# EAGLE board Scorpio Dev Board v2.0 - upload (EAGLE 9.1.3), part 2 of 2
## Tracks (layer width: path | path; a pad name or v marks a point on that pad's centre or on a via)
+5V  (via drill 0.48, 0.5, 0.8)
  Top 0.279: U1.73 59.42,28.71 v60.2,27.94
  Top 1.016: v85.85,20.19 85.85,19.68 90.04,15.49 JP12.1 JP12.2 JP12.3 JP12.4 | v5.59,87.63 56.46,87.63 57.98,86.19 57.98,80.45 68.45,69.98 73.53,69.98 79.63,63.88 79.63,61.72 79.76,61.59 82.96,61.59 84.84,59.72 U5.3 90.65,59.72 92.14,58.23 | X8.1 90.55,36.76 92.77,38.98 92.77,57.79 92.14,57.15 | 92.14,57.15 92.14,58.23 | R11.2 92.1,57.11 92.14,57.15 | JP14.2 92.33,55.88 92.33,58.42 | 92.33,58.42 92.14,58.23 | C12.1 92.33,60.68 92.33,58.42
  Bottom 0.61: v85.85,20.19 85.85,18.67 84.84,17.65 79.25,17.65 76.33,20.57 72.14,20.57 65.01,27.7 65.01,27.71 C9.1 62.09,27.94 v60.2,27.94
  Bottom 1.016: v85.85,20.19 85.85,35.79 X8.1 | JP5.1 6.22,82.68 3.68,85.22 R25.3 4.95,87.63 v5.59,87.63 5.59,90.3 6.1,90.81 8.64,90.81 9.91,92.08 JP20.2
AOUTL
  Top 0.254: U3.7 46.22,6.1 47.24,5.08 47.24,4.83 C39.1
AOUTR
  Top 0.254: U3.10 47.12,7.6 C38.1
BUTTON1
  Top 0.279: U1.29 31.33,32.22 21.34,22.22 JP15.12
  Bottom 0.305: 21.97,18.42 16.89,18.42
  Bottom 0.61: 21.97,18.42 22.61,19.05 22.61,21.59 21.97,22.22 JP15.12 | 16.89,18.42 16.19,19.11 15.91,19.39 15.24,19.39 12.29,19.39 R9.2 11.77,19.31 11.64,19.88 5.93,19.88 S2.3
BUTTON2
  Top 0.279: U1.34 32.89,29.71 21.59,18.42 19.43,18.42 JP15.13
BUTTON3
  Top 0.279: U1.87 71.98,35.72 73.28,34.42 74.04,34.42
  Top 0.305: 74.04,34.42 JP4.10 JP4.9
BUTTON4
  Top 0.279: U1.86 71.21,35.22 73.41,33.02 75.31,33.02 76.58,31.75
  Top 0.305: JP4.7 76.58,31.75
BUTTON5
  Top 0.279: U1.85 70.44,34.72 73.41,31.75
  Top 0.305: JP4.8 73.41,31.75
BUTTON6
  Top 0.279: U1.84 69.67,34.22 73.41,30.48 75.44,30.48
  Top 0.305: 75.44,30.48 JP4.5
BUTTON7
  Top 0.279: U1.83 68.9,33.72 73.41,29.21
  Top 0.305: JP4.6 73.41,29.21
CLKI  (via drill 0.5)
  Top 0.279: U1.71 55.62,24.89 57.15,23.37 57.28,23.37 | Y1.3 57.66,23.75 57.28,23.37 | v59.44,22.48 58.04,22.48 57.15,23.37 57.28,23.37
  Bottom 0.61: v59.44,22.48 62.61,22.48 65.53,19.56 JP10.1
CLKO  (via drill 0.5)
  Top 0.279: U1.72 56.12,25.67 56.39,25.4 v59.05,25.4
  Bottom 0.61: JP2.1 68.07,18.92 61.59,25.4 v59.05,25.4
D+  (via drill 0.5)
  Top 0.279: U1.77 63.14,30.71 64.52,29.34
  Top 0.406: 82.3,26.04 83.19,26.92 X1.D+
  Top 0.61: 64.52,29.34 72.9,20.96 80.39,20.96 80.77,21.34 v80.77,21.46 80.9,21.46 81.03,21.59 81.03,24.76 82.3,26.04
  Bottom 0.61: X8.3 86.68,41.4 82.68,41.4 81.15,39.88 81.15,21.84 v80.77,21.46
D-  (via drill 0.5)
  Top 0.279: U1.76 61.86,30.21 63.5,28.57
  Top 0.406: 83.57,25.4 83.57,25.65 84.19,26.27 X1.D-
  Top 0.61: 63.5,28.57 72.64,19.43 81.53,19.43 82.68,20.57 v82.68,21.46 82.68,24.51 83.57,25.4
  Bottom 0.61: X8.2 83.95,39.26 82.68,37.99 v82.68,21.46
DAC_FILT+
  Top 0.254: U3.6 45.47,5.6 C42.1
DAC_VQ
  Top 0.254: U3.5 40.69,4.62 40.26,4.19 40.26,4.17 C43.1
  Top 0.61: C43.1 C41.1
DEBUG_D+  (via drill 0.5)
  Top 0.254: X4.D+ 92.44,71.88 90.52,73.8 v90.39,73.8
  Bottom 0.406: v90.39,73.8 89.65,73.8 88.23,75.22 U11.15
DEBUG_D-  (via drill 0.5)
  Top 0.254: X4.D- 91.45,71.23 v90.42,72.26
  Bottom 0.406: U11.16 87.74,74.57 90.04,72.26 v90.42,72.26
DIPSW1
  Top 0.279: U1.27 29.79,33.22 21.34,24.76 JP15.10
DIPSW2
  Top 0.279: U1.28 30.56,32.72 21.34,23.5 19.43,23.5 JP15.9
ESP32_BOOT  (via drill 0.48, 0.5)
  Top 0.61: U6.25 96.14,81.92 94.87,83.19 v85.34,83.19 | v84.33,88.52 81.91,86.11 v81.91,84.2
  Top 0.813: v69.72,95.12 69.72,96.68 S4.2
  Bottom 0.61: v85.34,83.19 82.93,83.19 v81.91,84.2 | v84.33,88.52 v84.32,88.52 R30.1 80.86,88.69 77.85,88.69 74.97,91.57 70.1,91.57 69.72,91.95 v69.72,95.12
ESP32_CS  (via drill 0.48, 0.5)
  Top 0.279: U1.114 53.62,52.99 60.07,59.44 60.07,63.5 JP3.8
  Top 0.61: U6.29 93.47,87 v93.09,86.61 | v68.96,78.49 68.96,77.47 70.74,75.69 76.58,75.69 79.76,78.87 v81.28,78.87
  Bottom 0.61: JP3.8 58.8,67.31 68.96,77.47 v68.96,78.49 | v81.28,78.87 87.12,78.87 93.09,84.84 v93.09,86.61 93.09,89.41 R24.1
ESP32_EN  (via drill 0.5)
  Top 0.406: v77.09,93.22 76.64,93.22 75.56,92.13 75.56,89.53 75.06,89.03 71.37,89.03 70.17,87.82
  Top 0.61: U6.3 78.23,95.89 77.72,95.38 77.72,93.85 v77.09,93.22 | v69.09,81.28 69.09,86.79 70.17,87.82
  Bottom 0.61: R22.2 57.79,69.98 v69.09,81.28
  Bottom 0.813: R21.2 77.47,94.49 77.22,94.23 77.22,93.34 v77.09,93.22
ESP32_GPIO2  (via drill 0.48)
  Top 0.61: U6.24 94.36,78.89 93.57,78.11 v92.07,78.11
  Bottom 0.61: v92.07,78.11 93.6,79.63 R31.1
ESP32_HANDSHAKE  (via drill 0.5)
  Top 0.279: JP3.1 51.18,59.69 50.12,58.63 U1.121
  Top 0.61: U6.11 77.34,85.73 v77.28,85.66
  Bottom 0.305: JP3.1 52.45,63.5 | 52.45,63.5 | 52.45,66.55 52.45,63.5
  Bottom 0.61: 52.45,66.55 52.45,70.87 66.04,84.45 76.65,84.45 77.28,85.09 v77.28,85.66
ESP32_LED
  Top 0.61: U6.8 77.34,89.54 76.97,89.91 R23.1
ESP32_MISO  (via drill 0.48, 0.5)
  Top 0.279: U1.106 59.57,45.22 72.9,58.55 76.2,58.55 76.58,58.17 JP8.17
  Top 0.61: JP8.17 76.58,63.52 v71.9,68.2 | v75.6,78.49 77.25,78.49 79.16,80.39 v80.39,80.39 | v91.57,96.14 91.57,97.05 91.68,97.16 U6.37
  Bottom 0.406: 91.57,87.76 91.57,91.57
  Bottom 0.61: v75.6,78.49 75.6,75.58 71.9,71.88 v71.9,68.2 | v80.39,80.39 87,80.39 91.57,84.96 91.57,87.76 | 91.57,91.57 v91.57,96.14
ESP32_MOSI  (via drill 0.48, 0.5)
  Top 0.279: JP8.18 72.77,57.15 60.34,44.72 U1.105
  Top 0.61: v74.68,59.69 74.55,59.82 74.55,63.5 70.23,67.82 v70.23,68.2 | v73.8,78.49 73.8,82.69 73.79,82.71 v73.79,83.06 | v89.79,87.5 91.82,89.54 U6.31
  Bottom 0.61: JP8.18 74.68,57.79 v74.68,59.69 | v73.8,78.49 73.8,75.45 70.23,71.88 v70.23,68.2 | v89.79,87.5 87.5,87.5 85.6,85.6 81.53,85.6 78.99,83.06 v73.79,83.06
ESP32_MTDI
  Top 0.61: U6.14 76.98,81.92 76.21,81.15 R10.1
ESP32_RESET
  Top 0.279: U1.116 52.62,52.07 52.62,55.03 57.53,59.94 57.53,63.5 JP3.6
  Bottom 0.61: JP3.6 56.26,66.67 R22.1
ESP32_SCK  (via drill 0.48)
  Top 0.279: JP3.13 66.42,59.69 56.12,49.39 U1.109
  Top 0.61: v72.26,81.93 v72.26,78.49 | U6.30 92.71,88.27 89.92,85.47 v89.79,85.47
  Bottom 0.61: JP3.13 JP3.14 67.06,65.41 67.06,70.48 72.26,75.69 v72.26,78.49 | v89.79,85.47 85.98,81.66 72.53,81.66 v72.26,81.93
ESP32_TOUCH  (via drill 0.5, 0.8)
  Top 0.406: U6.9 79.52,88.14 72.26,88.14 v71.25,87.12
  Bottom 0.406: v71.25,87.12 68.45,87.12 v67.56,88.01
ESP32_VDD  (via drill 0.5)
  Top 0.61: 82.04,96.65 89.53,96.65 v90.04,96.14
  Top 0.813: U6.2 81.53,97.16 82.04,96.65 v82.04,96.27
  Top 0.914: C25.+ 75.92,97.16 U6.2
  Top 1.27: U7.2 U7.4 59.97,93.75 C33.1 64.24,93.75 64.52,93.47 74.17,93.47 75.67,94.97 C25.+
  Bottom 0.61: R30.2 C36.1 | R24.2 90.04,89.66 v90.04,96.14 90.04,96.39
  Bottom 0.813: C35.1 83.72,91.44 C36.1 | R21.1 82.04,95.29 v82.04,96.27
  Bottom 1.016: R21.1 82.43,93.85 C35.1 83.72,95.73 83.57,95.89 82.42,95.89 v82.04,96.27 82.57,95.73
ESP32_WAKE  (via drill 0.5)
  Top 0.279: JP3.5 56.26,59.69 54.36,57.79 52.12,55.55 U1.117
  Top 0.61: U6.10 73.28,87 70.61,84.33 v70.61,78.47
  Bottom 0.279: JP3.5 56.26,62.48 57.28,63.5 59.82,63.5 60.07,63.75 60.07,66.55
  Bottom 0.61: v70.61,78.47 70.61,77.34 60.07,66.8 60.07,66.55
FLASH_CS
  Top 0.279: U1.53 46.62,25.58 46.62,19.06 43.69,16.13 JP19.9
  Bottom 0.61: JP19.9 43.69,14.86 43.43,15.11 41.27,17.27 U2.1
FLASH_HOLD
  Top 0.279: JP19.5 48.77,14.73 49.12,15.08 49.12,25.58 U1.58 | JP19.5
FLASH_MISO
  Top 0.279: U1.48 44.12,21.26 40.51,17.65 40.39,17.65 38.48,17.65 37.34,16.51 37.34,13.21 JP19.14
  Bottom 0.305: 37.34,16 37.34,13.21 JP19.14
  Bottom 0.61: 37.34,16 37.34,19.43 40.39,22.48 U2.2
FLASH_MOSI
  Top 0.279: U1.69 54.62,23.36 60.2,17.78 60.2,14.48 60.2,13.21 JP7.2
  Bottom 0.61: U2.5 53.09,25.02 62.99,15.11 62.99,13.46 JP7.2
FLASH_SCK
  Top 0.279: JP19.6 47.5,13.21 47.5,15.24 48.62,16.36 48.62,25.58 U1.57
  Bottom 0.305: JP19.6 50.04,13.21 50.04,15.49 51.18,16.64
  Bottom 0.61: 51.18,16.64 51.18,23.24 50.67,23.75 U2.6
FLASH_WP
  Top 0.279: U1.47 43.62,21.65 40.64,18.67 38.23,18.67 36.07,16.51 JP19.15
  Bottom 0.61: JP19.15 36.07,18.54 | 36.07,18.54 36.07,20.19 39.62,23.75 U2.3 | R32.2 36.07,18.54
LCD_CS  (via drill 0.5)
  Top 0.279: U1.21 25.17,36.22 21.34,32.39 JP15.4
  Top 0.305: JP5.4 8.64,83.95 8.64,81.28
  Top 0.61: v7.87,76.33 8.64,77.09 8.64,81.28
  Bottom 0.305: JP15.4 22.48,32.39 22.99,32.89 22.99,35.81 22.61,36.2 16.89,36.2
  Bottom 0.61: 16.89,36.2 16.38,36.2 14.99,37.59 14.99,38.73 7.24,46.48 7.24,74.8 7.24,75.69 v7.87,76.33
LCD_RESET
  Top 0.279: U1.8 30.06,42.72 21.34,51.44 19.43,51.44 JP6.7
  Top 0.305: 13.72,80.9 13.72,83.95 JP5.8
  Top 0.61: 13.72,80.9 13.72,55.5 16.51,52.7 JP6.7
LCD_TE
  Top 0.279: U1.2 34.68,45.72 21.34,59.06 19.43,59.06 JP6.1
  Top 0.61: JP6.1 14.99,63.5 JP5.7
LED1
  Top 0.279: JP19.20 JP19.19 31.11,14.61 31.11,16.38 36.7,21.97 38.99,21.97 39.24,22.22 41.62,24.6 U1.43
  Top 0.305: R13.1 27.18,10.03 27.56,10.41 29.84,10.41 30.99,11.56
  Top 0.61: 30.99,11.56 JP19.20
LED2
  Top 0.279: U1.44 42.12,23.96 39.5,21.34 37.34,21.34 32.26,16.26 32.26,14.1 | JP19.18 32.26,13.21
  Top 0.305: 32.26,14.1 32.26,13.21 | R16.1 30.73,9.02 30.73,10.03 31.11,10.41 32.89,10.41 33.53,11.05 JP19.18
LED3  (via drill 0.48)
  Top 0.279: U1.45 42.62,23.19 | 42.62,23.19 | 42.62,23.19 40.01,20.57 37.85,20.57 33.53,16.26 JP19.17
  Top 0.305: R12.1 34.8,9.78 v34.8,10.54
  Bottom 0.305: v34.8,10.54 34.8,12.7 33.53,13.97 JP19.17
LED4
  Top 0.279: U1.46 43.12,22.42 40.26,19.56 37.85,19.56 34.8,16.51 34.8,13.21 JP19.16
  Top 0.305: R27.1 37.21,10.8 JP19.16
MCLR  (via drill 0.5)
  Top 0.279: U1.20 24.4,36.72 21.34,33.66 19.43,33.66 JP15.1
  Top 0.406: JP22.6 4.06,8.38 4.06,13.97 4.06,17.27 5.08,18.29 6.6,18.29 7.75,17.14 9.02,17.14 9.02,17.15
  Top 0.61: v11.68,30.1 11.68,22.99 9.27,20.57 R1.2 9.02,17.15
  Bottom 0.305: 16.89,31.11 19.05,31.11 19.43,31.5 19.43,33.66 JP15.1
  Bottom 0.61: v11.68,30.1 15.49,30.1 16.51,31.11 16.89,31.11
MCLR_IN
  Top 0.61: S1.3 5.82,11.28 6.61,12.07 R2.2 R1.1 11.91,14.35 C10.1
MCU_VDD  (via drill 0.5, 0.8)
  Top 0.279: 52.83,45.08 52.83,37.23 52.84,37.22 | v39.37,43.69 42.12,46.44 U1.137 | v51.94,45.72 50.55,45.72 49.62,46.64 U1.122 | U1.107 54.86,45.72 v54.74,45.72 | U1.88 v54.74,36.22 | U1.74 54.73,29.21 v54.1,29.85 | U1.33 38.11,30.21 38.48,29.85 v38.48,29.59 | U1.18 40.39,37.72 v41.27,36.83 | U1.55 47.62,29.21 v48.26,29.85 | U1.64 52.12,29.54 v51.82,29.85 | U1.41 40.62,29.06 v41.15,29.59
  Top 0.406: 57.75,48.86 57.28,48.39 57.28,47.37 55.63,45.72 54.86,45.72
  Top 0.61: v54.74,36.22 53.85,36.22 52.84,37.22 52.84,45.08 52.83,45.08 52.32,45.59 52.32,45.72
  Top 1.016: 57.75,48.86 68.07,59.18 v68.96,59.18 | v54.74,45.72 52.32,45.72 v51.94,45.72
  Bottom 0.61: C8.1 v54.74,45.72 | v51.94,45.72 C7.1 51.69,43.66 41.4,43.66 C6.1 | C1.1 41.55,36.55 v41.27,36.83 38.25,33.81 C2.1 38.25,29.82 v38.48,29.59 | v41.15,29.59 43.26,29.59 C4.1 47.01,28.6 v48.26,29.85 | R32.1 32.23,18.61 28.7,18.61 | 28.7,18.61 28.26,18.61 | v48.26,29.85 v51.82,29.85 52.2,30.23 C22.1 | C5.1 v48.26,29.85 | 54.12,29.83 54.12,35.59 v54.74,36.22 56.9,36.22 57.66,35.45 C3.1 | 28.7,18.61 28.13,18.61 26.29,16.76 25.78,16.76 21.21,12.19 L6.1 | C21.1 53.74,27.81 53.74,27.89 54.1,28.68 v54.1,29.85
  Bottom 0.813: v51.82,29.85 v54.1,29.85 54.12,29.83 | v39.37,43.69 41.17,43.69 C6.1
  Bottom 1.016: L3.1 71.65,62.38 68.96,59.69 v68.96,59.18 | 28.26,18.61 38.48,28.83 v38.48,29.59 v41.15,29.59
MISO4
  Top 0.279: JP8.12 72.77,49.53 64.96,41.72 U1.99
MOSI4
  Top 0.279: U1.104 61.11,44.22 66.17,49.28 72.77,55.88 75.31,55.88 JP8.15
N$1
  Top 0.61: R25.2 1.14,95.38 2.29,96.52 11.56,96.52 12.45,95.63 JP20.3
N$2
  Top 0.61: LED3.A R12.2
N$3
  Top 0.61: R23.2 72.03,90.81 LED6.A
N$6
  Top 0.61: C26.1 6.12,50.88 R19.2 C20.2
N$7
  Top 0.61: LED4.A 37.21,4.99 R27.2
  Top 1.016: LED4.A
N$8
  Bottom 0.61: R28.1 R29.1 20.03,38.14 JP13.1
N$11
  Bottom 0.406: R20.2 49.02,46.57 U8.2
N$12
  Bottom 1.016: JP23.1 84.58,10.17 X9.TSH
N$14
  Bottom 0.406: U8.1 50.29,51.44
  Bottom 0.61: 50.29,51.44 R4.2
N$15
  Bottom 0.406: U8.3 47.75,48.64 47.5,48.39 R7.2
N$17
  Top 1.016: R11.1 90.04,52.93 89.69,52.58 LED5.A
N$19
  Bottom 0.406: R8.1 37.72,57.28 39.24,55.75 46.02,55.75 U8.5
N$20
  Bottom 1.016: JP25.1 79.5,10.25 X9.RSH
N$21
  Bottom 0.406: U8.6 47.75,58.8 47.37,59.18 R17.1
N$22
  Bottom 0.61: X9.TIP 87.42,8.81 86.61,8 70.1,8 68.07,10.03 X3.3
N$23
  Bottom 0.61: X9.RING 77.25,9.65 70.74,9.65 70.06,10.33 X3.2
N$24  (via drill 0.48)
  Top 0.406: v84.2,73.91 83.03,73.91 C16.1
  Bottom 0.406: U11.17 v84.2,73.91
N$25
  Top 1.27: C28.1 48.64,93.07 U7.3 54.89,93.07 57.66,90.3 JP24.1
N$26
  Top 0.61: C18.2 5.56,57.28 C23.1 6.2,57.71 R15.2
N$27
  Top 0.61: R13.2 LED1.A
N$31
  Bottom 0.406: U8.7 49.02,60.07 48.26,60.83 45.47,60.83 45.21,60.58 45.21,57.66 44.7,57.15 41.02,57.15 R18.1
N$32
  Bottom 0.61: L3.2 74.65,64.69 C15.1
  Bottom 1.016: L3.2 L1.2
N$33
  Bottom 1.016: L5.2 17.19,12.55 L6.2 17.68,12.07 C17.1
N$34
  Top 0.61: X3.4 66.08,4.87 65.91,4.7 C40.1 59.03,2.92 58.27,2.16 R42.1
N$35
  Top 0.61: C39.2 50.65,2.39 R41.1 52.7,2.29 R42.2
N$38
  Top 0.61: C38.2 R39.2 54.73,9.53 R40.2
N$39
  Top 0.61: X3.5 64.07,7.68 63.37,6.98 C37.1 59.03,9.43 R40.1
N$46  (via drill 0.48)
  Top 0.406: v89.37,66.26 92.38,63.25 TX.C
  Bottom 0.406: R14.2 89.17,66.46 v89.37,66.26
N$63  (via drill 0.48)
  Top 0.406: v90.68,69.09 91.82,67.95 91.82,67.82 91.82,66.93 93.22,65.53 RX.C
  Bottom 0.406: R38.2 90.68,70.45 v90.68,69.09
N$80
  Top 0.61: LED2.A R16.2
OC2  (via drill 0.5)
  Top 0.279: U1.11 27.75,41.22 21.34,47.62 JP6.12
  Top 0.61: R19.1 10.95,48.9 v11.05,48.9
  Bottom 0.305: JP6.12 19.43,48.9 16.76,48.9
  Bottom 0.61: 16.76,48.9 v11.05,48.9
OC6  (via drill 0.5)
  Top 0.279: U1.6 31.6,43.72 21.34,53.98 19.43,53.98 JP6.5
  Top 0.61: R15.1 v10.92,55.25
  Bottom 0.61: JP6.5 v10.92,55.25
PGEC
  Top 0.279: U1.35 33.53,29.21 21.46,17.14 JP15.16
  Top 0.61: JP15.16 20.7,12.32 17.91,9.53 16.26,7.87 JP22.2
PGED  (via drill 0.5)
  Top 0.279: U1.36 34.05,28.71 25.4,20.07 v25.4,19.56
  Top 0.305: JP15.15 18.16,17.02
  Top 0.61: 18.16,17.02 18.16,15.24 18.16,12.45 13.84,8.13 13.84,6.48 JP22.3
  Bottom 0.406: v25.4,19.56 21.34,15.49 18.67,15.49 18.16,16 JP15.15
PMA0  (via drill 0.5)
  Top 0.279: U1.30 32.1,31.71 21.34,20.96 19.43,20.96 JP15.11
  Top 0.61: v14.35,34.42 14.86,34.42 15.62,33.66 15.62,24.89 18.16,22.35 JP15.11
  Bottom 0.305: JP5.3 8.64,83.95 8.64,87.38
  Bottom 0.61: v14.35,34.42 13.72,35.05 13.72,37.59 4.83,46.48 4.3,47.01 4.3,64.84 3.43,65.71 3.43,70.23 4.38,71.18 4.38,76.01 9.91,81.53 JP5.3 | JP20.4 15.11,94.11 15.11,90.93 12.32,88.14 9.4,88.14 8.64,87.38
PMCS1
  Top 0.279: JP8.10 72.77,46.99 66.5,40.72 U1.97
PMD0
  Top 0.279: U1.135 43.12,54.03 35.94,61.21 JP9.9
  Bottom 0.305: 16.26,81.15 16.26,83.95 JP5.10
  Bottom 0.61: JP9.9 34.42,60.71 25.02,60.71 23.88,61.85 23.88,63.63 21.46,66.04 19.94,66.04 16.26,69.72 16.26,81.15
PMD1
  Top 0.279: JP9.8 JP9.7 33.4,61.59 35.18,59.82 36.2,59.82 41.62,54.39 U1.138
  Bottom 0.61: JP5.9 17.53,75.95 22.92,70.55 25.78,70.55 25.78,70.48 28.96,67.31 32.77,67.31 33.4,66.67 JP9.8
PMD2  (via drill 0.5)
  Top 0.279: U1.142 39.62,50.29 33.65,56.26 32.38,56.26 28.32,60.33 JP9.3
  Top 0.305: 18.8,81.03 18.8,83.44 18.8,83.95 JP5.12
  Top 0.61: 18.8,81.03 18.8,80.65 v18.8,70.48
  Bottom 0.305: 27.05,66.42 27.05,63.5 JP9.3
  Bottom 0.61: v18.8,70.48 20.07,69.22 24.51,69.22 27.05,66.67 27.05,66.42
PMD3  (via drill 0.5)
  Top 0.279: JP9.2 27.05,63.5 27.05,60.33 31.75,55.63 33.27,55.63 39.12,49.78 U1.143
  Top 0.61: JP9.2 25.78,66.93 25.15,67.56 v25.15,72.39
  Bottom 0.61: JP5.11 20.07,75.95 23.62,72.39 v25.15,72.39
PMD4
  Top 0.279: JP9.1 25.78,60.33 31.11,54.99 32.89,54.99 38.62,49.26 U1.144
  Top 0.305: JP5.14 23.88,83.95 23.88,81.03
  Top 0.61: JP9.1 23.88,64.14 23.88,81.03
PMD5  (via drill 0.5)
  Top 0.279: U1.3 33.91,45.22 21.34,57.79 JP6.4
  Top 0.61: JP5.13 22.61,66.67 22.35,66.42 v22.35,62.74
  Bottom 0.61: v22.35,62.74 22.48,62.61 22.48,58.67 21.59,57.79 JP6.4
PMD6  (via drill 0.5)
  Top 0.279: U1.4 33.14,44.72 21.34,56.52 19.43,56.52 JP6.3
  Top 0.61: v19.3,62.87 20.83,64.39 20.83,76.2 v21.34,76.71
  Bottom 0.305: 23.88,81.03 23.88,83.95 JP5.16
  Bottom 0.61: v21.34,76.71 23.88,79.25 23.88,81.03 | JP6.3 16.51,57.79 15.75,58.55 15.75,61.98 16.64,62.87 v19.3,62.87
PMD7
  Top 0.279: U1.5 32.37,44.22 21.34,55.25 JP6.6
  Bottom 0.305: 37.21,60.58 37.21,66.42
  Bottom 0.61: 37.21,60.58 36.2,59.56 27.05,59.56 22.73,55.25 JP6.6 | JP5.15 25.15,78.23 27.05,76.33 27.05,72.39 30.23,69.22 34.42,69.22 37.21,66.42
PMD8
  Top 0.279: U1.128 46.62,51.44 46.62,59.17 44.83,60.96 44.83,63.5 JP9.16
  Top 0.305: 26.42,81.03 26.42,83.95 JP5.18
  Top 0.61: 26.42,81.03 26.42,77.09 35.94,67.56 42.93,67.56 43.56,66.93 JP9.16
  Bottom 0.61: JP20.7 22.61,89.15 24.07,87.69 26.61,87.69 27.69,86.61 JP5.18
PMD9  (via drill 0.5)
  Top 0.279: U1.127 47.12,59.94 46.1,60.96 JP9.17
  Top 0.61: JP5.17 27.69,77.6 36.58,68.71 44.32,68.71 44.83,68.2 v44.83,66.8
  Bottom 0.305: v44.83,66.8 44.83,63.5 JP9.17 | JP5.17 28.96,83.95 28.96,87.12
  Bottom 0.61: 28.96,87.12 27.43,88.65 25.4,88.65 25.15,88.9 JP20.8
PMD10  (via drill 0.5)
  Top 0.279: U1.125 48.12,59.17 48.64,59.69 JP9.19
  Top 0.305: JP5.20 28.96,83.95 28.96,81.03
  Top 0.61: v47.37,66.8 47.37,68.33 45.85,69.85 37.21,69.85 28.96,78.11 28.96,81.03
  Bottom 0.305: v47.37,66.8 47.37,63.5 JP9.19
  Bottom 0.61: JP5.20 30.1,85.34 30.1,87.25 27.69,89.66 JP20.9
PMD11
  Top 0.279: U1.124 48.62,58.4 49.91,59.69 49.91,63.5 JP9.20
  Top 0.61: JP5.19 30.23,78.74 37.97,70.99 47.5,70.99 48.64,69.85 JP9.20
  Bottom 0.305: JP5.19 31.5,83.95 31.5,87
  Bottom 0.61: 31.5,87 31.5,88.65 30.86,89.28 30.35,89.28 30.23,89.41 JP20.10
PMD12
  Top 0.279: JP3.10 62.61,63.5 62.61,59.69 54.62,51.7 U1.112
  Top 0.305: JP5.22 32.77,85.09 31.5,83.82 31.5,81.03
  Top 0.61: JP3.10 61.34,67.37 60.71,68.01 52.39,68.01 48.26,72.14 38.86,72.14 31.94,79.06 31.5,79.5 31.5,81.03
  Bottom 0.61: JP5.22 32.77,88.9 JP20.11
PMD13  (via drill 0.5)
  Top 0.279: JP3.9 61.34,59.69 54.12,52.47 U1.113
  Top 0.61: JP5.21 32.77,79.88 39.31,73.34 49.59,73.34 53.59,69.34 61.59,69.34 62.61,68.33 v62.61,66.8
  Bottom 0.305: JP3.9 62.61,63.5 v62.61,66.8 | JP5.21 34.04,83.95 34.04,87
  Bottom 0.61: 34.04,87 34.04,89.28 35.31,90.55 JP20.12
PMD14
  Top 0.279: U1.110 55.62,50.16 65.15,59.69 65.15,63.5 JP3.12
  Top 0.305: JP5.24 34.04,83.95 34.04,81.03
  Top 0.61: JP3.12 63.88,68.71 62.1,70.48 54.36,70.48 50.42,74.42 40.13,74.42 34.04,80.52 34.04,81.03
  Bottom 0.305: JP5.24 35.31,87.12 | 35.31,88.27 35.43,88.39
  Bottom 0.61: 35.31,87.12 35.31,88.27 | JP20.13 37.85,90.81 35.43,88.39
PMD15  (via drill 0.5)
  Top 0.279: U1.111 55.12,50.93 63.88,59.69 JP3.11
  Top 0.61: JP5.23 35.31,81.28 41.02,75.56 51.18,75.56 55.12,71.63 62.74,71.63 65.15,69.22 v65.15,68.45
  Bottom 0.305: JP3.11 65.15,63.5 v65.15,68.45 | JP5.23 36.58,83.95 36.58,87.12
  Bottom 0.61: JP20.14 40.39,91.44 36.58,87.63 36.58,87.12
PMRD
  Top 0.279: U1.13 26.21,40.22 21.34,45.08 JP6.14
  Bottom 0.279: JP6.14 20.7,45.72
  Bottom 0.305: 20.7,45.72 20.07,46.36 16.89,46.36 | JP5.6 11.18,83.95 11.18,81.15
  Bottom 0.61: 16.89,46.36 11.05,46.36 8.89,48.51 8.89,74.93 11.18,77.22 11.18,81.15
PMWR
  Top 0.279: U1.12 26.98,40.72 21.34,46.36 19.43,46.36 JP6.11
  Top 0.61: JP6.11 17.14,47.62 12.45,52.32 JP5.5
  Bottom 0.305: JP5.5 13.72,83.95 13.72,87.63
  Bottom 0.61: 13.72,87.63 14.35,88.27 18.16,88.27 20.07,90.17 JP20.6
PWM_OC2
  Top 0.406: C26.2 8.99,52.83 7.87,52.83 7.62,53.09 7.62,56.39 10.59,59.36 X6.TIP
PWM_OC6
  Top 0.61: C23.2 8.25,62.97 8.25,72.14 9.02,72.9 10.51,72.9 X6.RING
RA1
  Top 0.279: JP19.8 JP19.7 46.23,13.34 46.23,15.24 48.12,17.13 48.12,25.58 U1.56
RA9
  Top 0.279: JP1.2 27.18,11.94 27.05,12.07 27.05,15.24 35.18,23.37 35.56,23.37 37.72,23.37 39.62,25.27 U1.39
RA10
  Top 0.279: U1.40 40.12,24.88 37.97,22.73 35.56,22.73 28.32,15.49 JP1.1
RB4
  Top 0.279: U1.26 29.02,33.72 21.34,26.04 19.43,26.04 JP15.7
RB6
  Top 0.279: JP1.4 24,11.94 23.88,12.07 23.88,15.24 35.48,26.85 U1.37
RB7
  Top 0.279: U1.38 39.12,25.78 37.46,24.13 34.67,24.13 25.78,15.24 JP1.3
RB11
  Top 0.279: U1.50 45.12,20.45 40.68,16 40.39,16 39.88,15.49 39.88,13.21 JP19.12
RB12
  Top 0.279: U1.59 49.62,16.61 50.04,16.19 50.04,13.21 JP19.4
RB13
  Top 0.279: U1.60 50.12,17.32 51.31,16.13 JP19.3
RE8
  Top 0.279: U1.23 26.71,35.22 21.34,29.85 JP15.6
RE9
  Top 0.279: U1.24 27.48,34.72 21.34,28.57 19.43,28.57 JP15.5
REFCLKO1  (via drill 0.5)
  Top 0.254: U3.4 39.51,6.1 v39.12,5.71
  Top 0.279: U1.70 55.12,23.87 61.59,17.4 61.59,14.61 JP7.1
  Bottom 0.279: JP7.1 60.2,13.21 60.2,9.4 59.69,8.89 57.66,8.89
  Bottom 0.61: 57.66,8.89 55.75,6.98 52.7,6.98 51.43,5.71 v39.12,5.71
RF4
  Top 0.279: U1.90 71.5,37.22 72.01,37.22 73.66,37.22 JP8.2
RF5
  Top 0.279: JP8.1 75.31,38.1 72.77,38.1 72.39,37.72 U1.91
RG15
  Top 0.279: U1.1 35.57,46.22 21.46,60.33 JP6.2
RH4
  Top 0.279: U1.65 52.62,20.02 55.12,17.53 55.12,13.21 JP7.6
RH5
  Top 0.279: U1.66 53.12,20.92 56.39,17.65 JP7.5
RH6
  Top 0.279: U1.67 53.62,21.94 57.66,17.91 57.66,13.21 JP7.4
RH7
  Top 0.279: U1.68 54.12,22.71 58.93,17.91 JP7.3
RH8
  Top 0.279: U1.81 67.36,32.72 73.41,26.67
  Top 0.305: JP4.4 73.41,26.67
RH9
  Top 0.279: U1.82 68.13,33.22 73.41,27.94 75.44,27.94
  Top 0.305: 75.44,27.94 JP4.3
RH12
  Top 0.279: JP8.11 75.31,50.8 72.77,50.8 64.19,42.22 U1.100
RH13
  Top 0.279: U1.101 63.42,42.72 72.77,52.07 JP8.14
RH14
  Top 0.279: JP8.13 75.31,53.34 72.77,53.34 62.65,43.22 U1.102
RJ4
  Top 0.279: JP9.11 38.48,61.09 43.62,55.94 44.12,55.45 U1.133
RJ7
  Top 0.279: U1.134 43.62,54.68 37.21,61.09 37.21,63.5 JP9.10
RJ8
  Top 0.254: 21.34,52.7 JP6.8
  Top 0.279: 21.34,52.7 30.83,43.22 U1.7
RJ12
  Top 0.254: 21.34,50.17 JP6.10
  Top 0.279: 21.34,50.17 29.29,42.22 U1.9
RK0
  Top 0.279: JP15.2 21.46,34.92 23.88,37.22 U1.19
RK1
  Top 0.279: U1.51 45.62,20.07 41.15,15.59 JP19.11
RK2
  Top 0.279: U1.52 46.12,21.21 46.12,19.71 42.42,16 42.42,13.21 JP19.10
RK4
  Top 0.279: U1.92 69.6,38.22 69.84,38.22 71.62,38.22 72.77,39.37 JP8.4
RK5
  Top 0.279: JP8.3 75.31,40.64 72.77,40.64 70.85,38.72 U1.93
RK6
  Top 0.279: JP8.6 72.77,41.91 70.08,39.22 U1.94
RX_LED
  Bottom 0.406: U11.22 88.76,70.67 R38.1
SCK3
  Top 0.254: U3.2 42.29,7.1 42.29,9.53
  Top 0.279: U1.61 50.62,19.1 52.58,17.14 52.58,13.46 52.58,13.21 JP19.2
  Top 0.305: JP19.2 52.32,10.41 43.18,10.41 42.29,9.53
SCK4
  Top 0.279: JP8.9 75.31,48.26 72.77,48.26 65.73,41.22 U1.98
SCL1  (via drill 0.5)
  Top 0.279: JP8.5 75.31,43.18 72.77,43.18 69.31,39.72 U1.95
  Top 0.61: JP5.33 48.01,78.74 49.91,76.84 51.82,76.84 55.88,72.77 63.37,72.77 73.15,62.99 73.15,61.21 v73.28,61.09
  Bottom 0.61: v73.28,61.09 77.85,61.09 78.36,60.58 78.36,49.02 R5.2 78.23,47.37 78.23,42.55 77.6,41.91 JP8.5
SCL3
  Top 0.279: U1.80 66.59,32.22 73.41,25.4 75.44,25.4 JP4.1
SCL4
  Top 0.279: U1.16 23.37,38.72 22.99,38.72 22.48,38.72 22.22,38.72 21.99,38.72 JP6.15
  Bottom 0.61: JP6.15 20.87,39.84 R29.2
SD_CS  (via drill 0.5)
  Top 0.279: U1.22 36.74,35.7 26.51,35.7 21.92,31.11 19.43,31.11 JP15.3
  Top 0.61: X7.2 12.62,37 11.81,36.2 v11.81,35.56
  Bottom 0.61: v11.81,35.56 11.81,33.02 12.45,32.39 JP15.3
SD_MISO  (via drill 0.5)
  Top 0.279: U1.31 32.61,31.21 21.08,19.68 JP15.14
  Top 0.61: v5.97,42.8 6.27,42.5 X7.7
  Bottom 0.305: 16.76,20.96 19.43,20.96 JP15.14
  Bottom 0.61: 16.76,20.96 16.64,20.83 15.49,20.83 5.59,30.73 5.59,41.02 5.72,41.15 R3.1 5.71,42.54 v5.97,42.8
SD_MOSI  (via drill 0.5)
  Top 0.279: U1.25 28.25,34.22 21.34,27.31 JP15.8
  Top 0.61: v10.03,36.83 11.3,38.1 X7.3
  Bottom 0.305: 16.89,28.57 19.43,28.57 JP15.8
  Bottom 0.61: v10.03,36.83 10.03,28.96 10.41,28.57 16.89,28.57
SD_SCK
  Top 0.279: U1.14 25.49,39.72 21.34,43.81 19.43,43.81 JP6.13
  Top 0.61: X7.5 15.92,40.3 16.26,40.64 16.26,44.45 16.89,45.08 JP6.13
SDA1
  Top 0.279: U1.96 68.54,40.22 72.77,44.45 JP8.8 JP8.7
  Bottom 0.305: JP5.36 51.82,83.95 51.82,81.15 | 49.91,66.55 49.91,60.2
  Bottom 0.406: 49.91,60.2 51.43,58.67 58.42,58.67
  Bottom 0.61: 68.2,44.45 JP8.8 | 58.42,58.67 68.2,48.9 68.2,44.45 | 51.82,81.15 51.82,78.74 49.91,76.84 49.91,66.55 | R6.2 68.2,44.45
SDA3
  Top 0.279: U1.79 65.82,31.71 73.41,24.13 JP4.2
SDA4
  Top 0.279: U1.15 24.67,39.22 21.34,42.55 JP6.16
  Bottom 0.305: R28.2 24.13,41.4 22.99,42.55 JP6.16
SDO3  (via drill 0.5)
  Top 0.254: U3.1 39.75,7.6 39.75,8
  Top 0.279: U1.49 44.62,20.83 40.81,17.02 39.62,17.02 38.61,16 JP19.13
  Top 0.61: v39.88,10.29 39.88,8.13 39.75,8
  Bottom 0.305: JP19.13 39.88,13.21 v39.88,10.29
SPI2_CS
  Top 0.279: U1.10 28.52,41.72 21.34,48.9 19.43,48.9 JP6.9
SPI4_CS
  Top 0.279: JP8.16 72.77,54.61 61.88,43.72 U1.103
SQICLK
  Top 0.279: U1.129 46.12,50.8 46.12,58.65 43.56,61.21 JP9.15
  Bottom 0.305: R17.2 43.81,62.23 JP9.15
SQID0  (via drill 0.5)
  Top 0.279: JP9.4 29.59,63.5 29.59,60.45 v32.19,57.85 33.02,57.02 34.04,57.02 40.12,50.94 U1.141
  Bottom 0.406: v32.19,57.85 34.03,57.85 R8.2
SQID1  (via drill 0.5)
  Top 0.279: JP9.5 30.86,61.04 33.48,58.42 34.29,58.42 v39.05,53.66 40.62,52.09 U1.140
  Bottom 0.406: v39.05,53.66 39.05,47.18 40.64,45.59 46.35,45.59 R20.1
SQID2  (via drill 0.5)
  Top 0.279: JP9.6 32.13,63.5 32.13,61.21 34.29,59.06 35.18,59.06 v40.64,53.59 41.12,53.11 U1.139
  Bottom 0.406: R7.1 40.64,49.01 v40.64,53.59
SQID3
  Top 0.279: U1.130 45.62,57.76 42.29,61.09 42.29,63.5 JP9.14
  Bottom 0.305: 42.29,61.09 42.29,63.5 JP9.14
  Bottom 0.406: R18.2 41.28,60.07 42.29,61.09
SRAM_CS  (via drill 0.5)
  Top 0.279: JP3.7 58.8,59.56 v54.26,55.02 53.12,53.88 U1.115
  Bottom 0.61: R4.1 55.02,51.45 55.02,54.26 v54.26,55.02
SS3  (via drill 0.48)
  Top 0.254: U3.3 43.05,6.6 43.05,9.14 43.69,9.78 45.73,9.78 v45.97,9.54
  Top 0.279: U1.62 51.12,20 53.85,17.27 JP19.1
  Bottom 0.279: JP19.1 55.12,13.21
  Bottom 0.305: 55.12,13.21 55.12,10.67 53.99,9.54 v45.97,9.54
TFT_BL
  Top 0.279: JP3.2 52.45,63.5 52.45,59.69 50.62,57.86 U1.120
  Bottom 0.305: JP5.40 54.36,83.95 54.36,81.41
  Bottom 0.61: JP20.15 42.93,90.55 43.31,90.17 54.23,90.17 55.63,88.77 55.63,86.49 JP5.40 | JP3.2 51.18,72.52 54.36,75.69 54.36,81.41
TP_IRQ
  Top 0.279: JP9.18 46.1,64.64 47.37,63.37 47.37,61.47 47.62,61.22 47.62,56.64 U1.126
  Bottom 0.61: JP5.35 50.67,82.55 50.67,80.77 48.26,78.36 48.26,69.85 46.1,67.69 JP9.18
TP_RESET
  Top 0.279: U1.131 45.12,57.24 41.02,61.34 JP9.13
  Bottom 0.305: JP9.13 39.75,63.5 39.75,66.42 | 46.74,81.03 46.74,83.95 JP5.34
  Bottom 0.61: 46.74,81.03 46.74,70.87 44.32,68.45 41.66,68.45 39.75,66.55 39.75,66.42
TP_WAKE
  Top 0.279: U1.132 44.62,56.22 39.75,61.09 39.75,63.5 JP9.12
  Bottom 0.305: 41.66,87.12 41.66,81.03
  Bottom 0.61: JP9.12 38.48,67.69 41.66,70.87 41.66,81.03 | JP5.38 53.09,86.74 52.32,87.5 41.91,87.5 41.66,87.25 41.66,87.12
TX_LED
  Bottom 0.406: U11.23 87.46,70.02 87.88,69.6 87.88,68.29 R14.1
U4RX  (via drill 0.5)
  Top 0.279: JP3.3 53.72,59.69 51.12,57.09 U1.119
  Top 0.61: U6.34 v95.63,93.34
  Bottom 0.406: 82.74,75.63 82.55,75.44 82.55,72.14 81.66,71.25 81.66,67.56 80.87,66.77 U11.1 72.23,66.77 71.56,66.1 | 82.74,75.63 82.93,75.82 | 82.74,75.63
  Bottom 0.61: JP3.3 53.72,60.96 54.36,60.33 67.06,60.33 68.71,61.98 68.71,63.25 70.93,65.47 71.56,66.1 | 82.93,75.82 83.69,76.58 88.39,76.58 95.76,83.95 95.76,93.22 v95.63,93.34
U4TX  (via drill 0.48)
  Top 0.279: U1.118 51.62,56.32 54.99,59.69 54.99,63.5 JP3.4
  Top 0.61: v93.34,94.62 U6.35
  Bottom 0.406: 81.53,77.6 81.53,73.15 80.77,72.39 80.77,69.85 80.29,69.37 U11.5
  Bottom 0.61: JP3.4 53.72,69.72 66.67,82.68 69.72,82.68 72.26,80.14 77.85,80.14 78.61,79.38 78.61,78.36 79.38,77.6 79.5,77.6 81.41,77.6 81.53,77.6 87.76,77.6 94.74,84.58 94.74,91.44 93.34,92.84 v93.34,94.62
USB_ID
  Top 0.279: U1.78 64.42,31.21 65.53,30.1
  Top 0.406: 79.39,27.57 X1.ID
  Top 0.61: 65.53,30.1 71.5,24.13 73.41,22.22 77.85,22.22 79.12,23.5 79.12,27.31 79.39,27.57
VBUS  (via drill 0.48)
  Top 0.406: 89.28,69.72 90.14,70.58 X4.VBUS | X1.VBUS 92.3,25.62 v91.19,24.51 | TX.A RX.A
  Top 0.61: TX.A 98.81,63.25 98.81,53.98 98.17,53.34 JP14.3
  Top 0.813: 86.11,68.45 85.05,68.45 C29.1
  Top 1.016: JP24.2 61.34,90.17 61.34,79.88 69.09,72.14 75.69,72.14 v75.82,72.01 75.95,72.14 83.44,72.14 85.07,70.51 C29.1 | v89.79,67.69 89.79,67.82 89.15,68.45 | 86.11,68.45 89.15,68.45 | 89.15,68.45 89.15,69.6 89.28,69.72
  Bottom 0.406: U11.4 76.85,68.72 76.84,68.71 76.58,68.71 75.82,69.47 v75.82,72.01 | U11.20 84.16,71.97 82.66,70.47 82.66,65.3
  Bottom 0.61: C31.1 C30.1 87.02,64.52 82.78,64.52 82.66,64.39
  Bottom 1.016: 92.46,58.67 92.46,63.5 92.46,65.28 90.98,66.75 90.98,66.77 90.06,67.69 v89.79,67.69 | 82.66,65.3 82.66,64.39 82.66,63.12 82.66,60.2 84.18,58.67 92.46,58.67 | 92.46,58.67 92.84,58.67 92.84,52.96 92.96,52.83 | v91.19,24.51 91.19,30.48 92.46,31.75 92.46,52.07 92.46,52.32 92.96,52.83 | 92.96,52.83 93.6,53.47 96.01,53.47 JP14.3
VDD  (via drill 0.48, 0.5)
  Top 0.254: U3.9 43.94,7.11 43.69,7.37 43.69,8.38 44.07,8.76 v44.58,8.76
  Top 0.61: JP18.1 16.89,37.47 16.26,38.1 16.26,38.73 15.79,39.2 X7.4 10.37,39.2 v8,36.83 | 83.69,17.65 77.22,17.65 75.82,16.26 65.53,16.26 64.33,17.46 64.33,18.1 64.33,18.58 C11.1 62.99,18.67 61.85,19.81 61.85,21.13 Y1.4 | JP22.5 8.64,8.63 R2.1
  Top 1.016: JP16.4 JP16.3 JP16.2 JP16.1 90.04,11.43 83.82,17.65 83.69,17.65 83.69,19.18 v83.57,19.3 | v5.21,22.86 6.98,22.86 8.13,24 8.13,30.86 8.13,36.7 v8,36.83 | 83.69,57.4 U5.4 80.72,52.63 C13.1 | 83.69,57.4 U5.2 | v83.69,55.5 83.69,57.4 | v23.75,3.18 9.91,3.18 8.64,4.45 JP22.5
  Bottom 0.305: 72.26,40.64 78.1,40.64 78.61,40.64 | C19.1 47.35,17.25 46.1,16 45.47,16 44.96,15.49 44.96,13.84 44.32,13.21 42.67,13.21 42.42,12.95 42.42,9.65 42.04,9.27 41.66,8.89
  Bottom 0.61: v5.21,22.86 3.68,21.34 3.68,15.37 4.19,14.86 | 4.19,14.86 5.59,13.46 | 68.2,40.64 72.26,40.64 | 68.2,40.64 62.99,40.64 62.09,41.54 62.09,49.42 54.91,56.6 52.06,56.6 C24.1 51.02,56.22 U8.8 | U2.7 U2.8 49.4,19.05 48.37,18.02 47.36,18.02 C19.1 | R6.1 68.2,40.64 | 4.19,14.86 | R5.1 81.92,47.45 79.72,45.25 | 36.32,3.18 36.32,5.87 C45.1 36.42,6.6 C44.1 36.93,8.89 41.15,8.89 | 41.15,8.89 41.66,8.89 | 41.15,8.89 44.45,8.89 v44.58,8.76
  Bottom 0.813: R3.2 8.51,38.1 8,37.59 v8,36.83
  Bottom 1.016: JP16.1 90.04,8.76 87.88,6.6 85.85,6.6 84.96,5.71 84.96,3.68 83.95,2.67 80.65,2.67 79.25,4.06 79.25,5.84 78.49,6.6 60.83,6.6 60.13,5.91 58.1,3.87 57.4,3.18 37.34,3.18 36.32,3.18 v23.75,3.18 | v83.57,19.3 80.01,19.3 78.95,20.36 78.95,40.64 | v83.69,55.5 81.56,55.5 81.92,55.14 | R9.1 11.81,14.86 10.41,13.46 9.14,13.46 | R5.1 81.92,55.14 | 81.92,55.14 79.84,57.22 79.84,62.75 L1.1 | 5.59,13.46 8.64,13.46 9.14,13.46 | JP22.5 8.64,9.02 8.95,9.34 | 8.95,9.34 9.14,9.53 14.83,9.53 L5.1 | 8.95,9.34 8.95,13.27 9.14,13.46 | 78.95,40.64 78.61,40.64 | 79.72,45.25 79.72,41.4 78.95,40.64
VSS  (via drill 0.48, 0.5, 0.8)  (26 unrouted)
  Top 0.254: U3.8 48.9,6.6 49.02,6.48 | Y1.2 63.96,24.81 63.75,25.02 60.32,25.02 | 57.53,24.38 59.69,24.38 60.32,25.02 | 66.67,21.84 66.04,22.48 60.83,22.48 59.69,21.34 58.93,21.34 58.42,21.84 | 60.32,25.02 60.32,25.78 59.69,26.42 57.4,26.42 | U1.32 45.95,30.71 46.35,31.11
  Top 0.279: U1.17 40.26,38.22 41.27,39.23 41.27,40 | 47.12,28.45 47.12,30.35 46.35,31.11 | U1.63 51.62,28.26 50.29,29.59 50.29,32 | U1.123 49.12,46.96 47.88,45.72 45.85,45.72 43.56,45.72 42.62,46.66 U1.136 | v55.88,30.48 55.88,30.23 56.39,29.71 U1.75 60.58,29.71 61.35,28.94 | v54.74,38.86 54.74,38.48 56.5,36.72 U1.89 | 47.12,28.45 41.61,28.45 41.12,27.96 U1.42 | 57.4,26.42 56.9,26.92 56.9,27.43 | 59.69,21.34 59.69,20.45 63.63,16.51 63.63,13.08 63.63,12.83 64.01,12.45 69.09,12.45 69.85,13.21 69.85,14.61 | U1.54 47.12,28.45 | U1.108 58,46.23 59.44,46.23 60.07,46.86 60.07,47.62 60.71,48.26
  Top 0.406: X1.GND 90.39,28.22 89.6,29.02 89.47,29.02 | 92.2,74.33 92.28,74.33 93.42,73.18 X4.GND | 63.63,13.08 62.99,12.45 | 49.02,6.48 52.19,6.48 | C42.2 46.12,0.51 58.04,0.51 | C16.2 77.22,74.3 v77.09,74.17 | v88.14,72.14 88.14,75.59 88.26,75.72 | v84.07,67.18 82.07,67.18 | C29.2 78.74,69.09 v77.09,70.74
  Top 0.61: X7.6 7.24,41.4 5.84,40 | 5.84,40 5.84,31.11 4.83,30.1 4.72,30.2 X7.S1 3.68,30.2 3.68,23.88 | 2.29,46 1.93,46 1.14,45.21 1.14,41.02 2.16,40 5.84,40 | 3.68,23.88 3.68,22.38 S2.1 2.62,19.99 3.05,19.56 3.05,15.37 2.03,14.35 v2.03,13.59 1.29,12.85 S1.1 | 3.68,23.88 v2.03,23.88 | C11.2 66.67,18.67 66.67,21.84 | v38.86,1.02 40.72,1.02 C43.2 | v74.55,85.74 74.55,84.72 75.1,84.17 76.06,83.94 R10.2 | JP22.4 11.18,9.02 12.7,10.54 13.33,10.54 13.97,11.18 13.97,16.51 13.1,17.38 C10.2 | 44.96,1.17 C42.2 | 52.19,6.48 R39.1 55.4,5.33 C40.2 C37.2 | 67.18,90.68 v66.8,90.68 | 72.42,98.45 72.77,98.81
  Top 0.813: 88.52,91.59 U6.1.1 | 77.98,98.81 74.04,98.81 | 53.47,98.42 53.85,98.81 | C33.2 61.98,96.88
  Top 0.914: v88.52,94.74 88.52,91.59 | U6.38 U6.1 78.36,98.42 77.98,98.81 68.45,98.81 | 86.55,86.68 82.93,83.06 U6.15 82.93,77.47 | S4.1 61.87,96.77 C33.2
  Top 1.016: JP17.2 JP17.3 | X7.S3 3.94,46.06 X7.S2 2.29,46 1.14,47.14 1.14,50.65 C20.1 C18.1 1.17,66.7 2.29,67.82 X6.SLEEVE | 89.47,29.02 88.71,29.78 v88.2,29.78 88.01,29.59 83.82,29.59 83.57,29.85 83.57,42.87 84.45,43.76 X8.4 85.94,44.65 85.94,52.56 LED5.C | 46.35,31.11 47.62,32.39 49.91,32.39 | 50.29,32 49.91,32.39 | 45.85,45.72 45.85,41.02 44.83,40 41.27,40 | 17.53,90.81 45.09,90.81 45.47,91.19 JP20.16 45.47,96.39 46.84,97.77 C28.2 48.92,98.04 51.79,98.04 U7.1 52.73,97.69 53.47,98.42 | 33.4,1.37 35.31,1.37 LED4.C 37.57,1.02 v38.86,1.02 | v20.32,1.27 20.42,1.37 24.89,1.37 | JP20.5 17.53,90.81 | U5.1 85.95,54.13 LED5.C | LED5.C C13.2 | v71.5,4.45 73.91,6.86 | 73.91,6.86 82.42,6.86 X9.SLEEVE | 49.91,32.39 55.37,32.39 55.88,31.88 v55.88,30.48 | v58.93,47.62 60.06,47.62 60.71,48.26 71.51,59.07 71.51,59.18 v71.63,59.18 71.63,62.23 v68.58,65.28 | 82.93,77.47 84.68,75.72 88.26,75.72 90.81,75.72 92.2,74.33 | C29.2 82.07,67.18 82.07,65 v85.09,61.98 | JP5.2 7.24,85.09 6.35,85.09 3.68,82.42 R25.1 | 73.91,6.86 73.91,9.57 X3.1 | JP20.1 7.37,91.44 8,90.81 17.53,90.81
  Top 1.27: 64.52,98.81 68.45,98.81 72.77,98.81 | 64.52,98.81 61.98,98.81 | 53.85,98.81 61.98,98.81 | 61.98,98.81 61.98,96.88 62.08,96.77 S4.1 64.23,98.52 64.52,98.81 | C25.- 72.42,98.45 | 24.89,1.37 LED1.C LED2.C | LED2.C | LED2.C 33.4,1.37 | LED3.C | LED3.C LED4.C 40.56,1.37 C43.2 C41.2 44.96,1.17 | C42.2 47.4,1.17 47.75,1.52 R41.2 | v85.09,61.98 C12.2 | LED6.C 67.18,90.68
  Top 2.032: U6.1.1 87.82,90.89 87.82,88.65 86.55,87.38 86.55,86.68 | U6.1.1 87.95,94.17 88.01,94.23 | U6.1.1 87.9,91.06 85.22,91.06 | U6.1.1 90.13,91.02 90.3,91.19
  Bottom 0.406: U11.7 77.67,70.67 77.09,71.25 | 77.09,71.25 v77.09,74.17 | U11.18 87.64,73.27 88.14,72.77 v88.14,72.14 88.14,71.63 87.83,71.32 U11.21 84.65,71.32 84.33,70.99 84.33,68.96 | 84.33,68.96 84.57,68.72 U11.25 U11.26 84.46,68.07 84.33,68.2 84.33,68.96 | 84.33,68.96 84.07,68.71 v84.07,67.18 | v77.09,70.74 77.09,71.25
  Bottom 0.61: U8.4 46.48,53.72 | 46.48,53.72 46.48,54.23 45.85,54.86 36.32,54.86 35.56,54.1 35.56,43.81 38.58,40.79 C6.2 | v58.93,47.62 57.66,46.35 57.66,42.42 56.03,40.79 C8.2 | C24.2 52.02,53.72 46.48,53.72 | C45.2 C44.2 | C22.2 52.2,40.72 | C30.2 85.45,61.62 v85.09,61.98 | C15.2 74.29,68.3 74.29,72.52 75.95,74.17 v77.09,74.17 | 65.41,85.74 v74.55,85.74
  Bottom 1.016: C3.2 56.51,31.65 55.88,31.01 v55.88,30.48 55.88,29.72 56.64,28.96 56.64,27.71 C21.2 | v54.74,38.86 C8.2 | JP22.4 11.18,1.14 | 11.18,1.14 20.19,1.14 v20.32,1.27 20.95,1.91 20.95,7.62 20.93,7.64 20.93,9.27 C17.2 | v6.73,1.65 7.24,1.14 | 7.24,1.14 11.18,1.14 | X3.1 73.77,11.41 76.45,14.1 76.45,15.37 | 76.45,15.37 v74.04,17.78 | 76.45,15.37 76.45,16 82.04,16 | 82.04,16 JP11.1 | 82.04,16 86.61,16 88.26,17.65 88.26,29.72 v88.2,29.78 | 65.02,90.55 65.02,98.68 v65.15,98.81 | 52.2,40.72 51.95,40.79 | v88.52,94.74 87.63,93.85 C35.2 86.72,91.44 C36.2 | C31.2 89.51,61.59 87.15,61.59 C30.2 | 65.02,90.55 65.02,86.36 v63.63,84.96 | v66.8,90.68 65.15,90.68 65.02,90.55 | 65.41,85.74 64.4,85.74 v63.63,84.96 | JP5.39 61.34,82.68 v63.63,84.96 | S1.1 1.29,2.9 3.05,1.14 7.24,1.14
  Bottom 1.27: 97.16,77.72 97.41,77.98 R31.2 97.28,79.76 97.28,81.53 | 51.95,40.79 C8.2 | C7.2 51.82,40.79 C6.2
  pour Bottom (isolate 0.406): 0,99.95 0,0 99.95,0 99.95,99.95
  pour Top (isolate 0.406): 0,99.95 0,0 99.95,0 99.95,99.7 98.55,99.95 98.81,99.7

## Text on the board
tPlace: VSS | 5V | VO | RS | RW | EN | D8 | D9 | D10 | D11 | D12 | D13 | D14 | D15 | BL | VSS | BOOT | HD44780 LCD | ESP32 | VSS | CS | RD | RST | D0 | D2 | D4 | D6 | D8 | D10 | D12 | D14 | RST | SDA | WAK | BL | 5V | DC | WR | TE | D1 | D3 | D5 | D7 | D9 | D11 | D13 | D15 | SCL | IRQ | PEN | VSS | 16-bit TFT LCD with touch | 44.1khz PWM | X4 | DEBUG | RA5 / G15 | RE3 / RE4 | G13 / RE2 | G14 / G12 | RE1 / RE1 | RJ7 / RE0 | RJ5 / RJ6 | RA7 / RJ4 | RG0 / RA6 | RK7 / RG1 | RF0 / RF1 | RD6 / RD7 | RD4 / RD5 | RJ2 / RJ3 | RJ0 / RJ1 | D12 / D13 | RD2 / RD3 | RD1 / RD1 | POWER | C14 / C13 | RE6 / RE5 | PIC32MZ2048EFH144 Scorpio v2.0 | RD0 / H15 | RC1 / RE7 | H14 / H13 | RJ9 / RJ8 | by Aidan Mocke 2019-01-18 | H12 / D11 | J10 / J12 | HOST | SPI SD | D10 / RD9 | RC3 / RC2 | A15 / A15 | RG6 / RC4 | A14 / RK6 | RG8 / RG7 | JLCJLCJLCJLC | RK5 / RK4 | X8 | I2C4 | X7 | pullups | RF5 / RF4 | RA4 / RA4 | MCL / RK0 | RA3 / RA2 | RA0 / RG9 | DEVICE | H11 / H10 | RE9 / RE8 | BUTTON | 1 | RH9 / RH8 | X1 | RB4 / RB5 | RF8 / RF2 | J13 / J11 | Thanks to Bryn | J15 / J14 | RB2 / RB3 | for whatever | 5V | RESET | RB0 / RB1 | RB7 / RB6 | A10 / RA9 | RH0 / RH0 | RH2 / RH1 | RB8 / RH3 | B10 / RB9 | RK1 / B11 | RK3 / RK2 | RA1 / RA1 | F12 / F13 | B13 / B12 | B15 / B14 | RH5 / RH4 | RH7 / RH6 | D15 / D14 | CLKI | CLKO | DAC OUT | 3V3 | GND | * | ICSP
